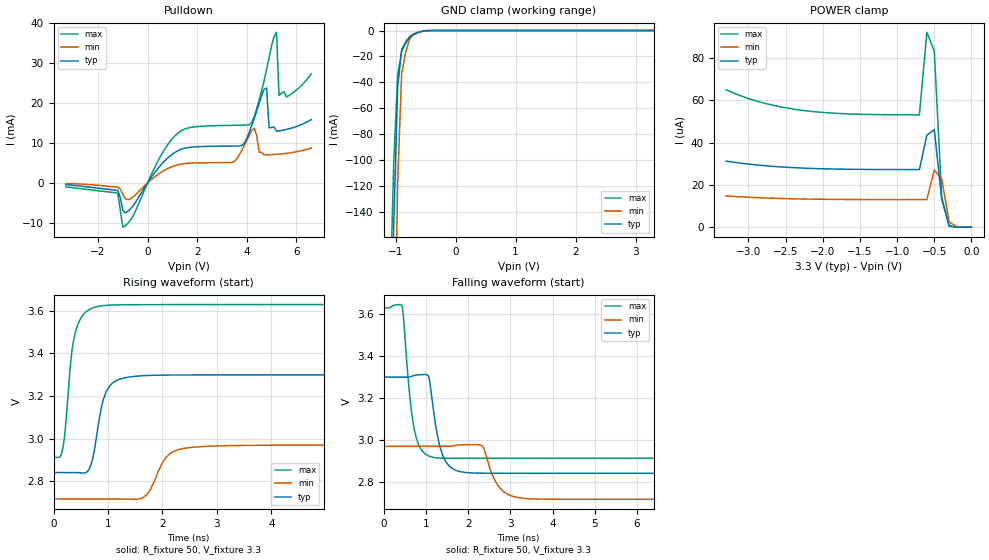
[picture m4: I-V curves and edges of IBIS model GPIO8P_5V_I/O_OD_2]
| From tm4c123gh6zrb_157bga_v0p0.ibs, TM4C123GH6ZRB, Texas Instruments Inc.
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|   Model Cell GPIO8P_5V_I/O_OD_2
[Model]   GPIO8P_5V_I/O_OD_2
Model_type   I/O_open_drain
Polarity   Inverting
Enable   Active-Low
Vinl =  0.8
Vinh =  2
Cref =  15.0000pF
Rref =  100.0000M
Vref =  0V
Vmeas =  1.65
C_comp   4.711578p   4.034737p   5.423069p
[Model Spec]
Vinl   0.8   0.8   0.8
Vinh   2   2   2
[Temperature Range]   25   125   -40
[Voltage Range]   3.3   2.97   3.63
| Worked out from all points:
|   slope of the pulldown table from 0 to 0.495 V, typ, clamps not added: 118 ohm
|   GND clamp passes 1 mA (typ) near -0.59 V on its own axis
|   rising waveform, R_fixture 50, V_fixture 3.3: 20-80 % time 209ps typ, 304ps min, 170ps max; typ from 2.84 V to 3.3 V
|   falling waveform, R_fixture 50, V_fixture 3.3: 20-80 % time 252ps typ, 337ps min, 213ps max; typ from 3.3 V to 2.84 V
| Nom Voltages:
|   VDDC=1.2, VDD=3.3, GND=0
| Min Voltages:
|   VDDC=1.08, VDD=2.97, GND=0
| Max Voltages:
|   VDDC=1.32, VDD=3.63, GND=0
[POWER_clamp]
|   voltage   I(typ)   I(min)   I(max)
-3.3V     31.22uA    14.76uA    64.95uA
-3.1V     30.25uA    14.33uA    62.09uA
-2.8V     29.13uA    13.84uA    58.77uA
-2.3V     27.98uA    13.34uA    55.36uA
-1.7V     27.4uA     13.1uA     53.62uA
-700mV    27.24uA    13.03uA    53.12uA
-600mV    43.52uA    13.03uA    92.14uA
-500mV    46.16uA    27.05uA    83.3uA
-400mV    13.21uA    22.74uA    13.98uA
-300mV    630.7nA    2.501uA    480.9nA
-200mV    23.21nA    190.8nA    10.65nA
0V        660.4pA    10.19nA    564.9pA
[Pulldown]
|   voltage   I(typ)   I(min)   I(max)
-3.3V     -450.7uA   -192.2uA   -1.006mA
-1.2V     -1.893mA   -1.109mA   -2.697mA
-1V       -6.866mA   -2.892mA   -11.1mA
1.2V      7.958mA    4.478mA    12.33mA
3.5V      9.211mA    5.381mA    14.4mA
4.2V      14.36mA    13.04mA    15.06mA
4.5V      19.92mA    7.668mA    20.83mA
4.8V      23.73mA    7.004mA    28.42mA
4.9V      13.75mA    7.03mA     31.35mA
5.2V      12.91mA    7.14mA     37.68mA
5.3V      13mA       7.19mA     21.9mA
6.6V      15.82mA    8.714mA    27.27mA
[GND_clamp]
|   voltage   I(typ)   I(min)   I(max)
-3.3V     -16.3A     -15.26A    -17.13A
-1.1V     -340.4mA   -570.5mA   -222.8mA
-1.033V   -152.7mA   -296.8mA   -103.3mA
-966.7mV  -44.18mA   -117.7mA   -34.4mA
-900mV    -14.77mA   -33.12mA   -16.14mA
-833.3mV  -8.752mA   -16.68mA   -9.833mA
-766.7mV  -4.716mA   -6.551mA   -5.563mA
-700mV    -2.657mA   -2.741mA   -3.333mA
-566.7mV  -672.8uA   -727.2uA   -724.4uA
-433.3mV  -51.87uA   -90.8uA    -37.79uA
3.3V      660.4pA    5.308uA    422.7pA
[Ramp]
| variable   typ   min   max
dV/dt_f 0.28269897/0.25386606n 0.15654957/0.33829046n 0.43992818/0.21519855n
dV/dt_r 0.38699946/0.53401128n 0.23880101/0.85366195n 0.55927105/0.38819382n
R_load = 50
[Rising Waveform]
R_fixture = 50
V_fixture = 3.3
V_fixture_min = 2.97
V_fixture_max = 3.63
|   time   V(typ)   V(min)   V(max)
0s        2.841V     2.717V     2.912V
178.1ps   2.841V     2.717V     2.965V
341.5ps   2.841V     2.717V     3.419V
428.4ps   2.841V     2.717V     3.523V
687.2ps   2.877V     2.717V     3.61V
833.7ps   3.083V     2.717V     3.622V
1.166ns   3.274V     2.717V     3.628V
2.143ns   3.299V     2.931V     3.63V
2.818ns   3.299V     2.964V     3.63V
20.12ns   3.3V       2.97V      3.63V
[Falling Waveform]
R_fixture = 50
V_fixture = 3.3
V_fixture_min = 2.97
V_fixture_max = 3.63
|   time   V(typ)   V(min)   V(max)
0s        3.3V       2.97V      3.63V
436.2ps   3.3V       2.97V      3.639V
720.2ps   3.308V     2.97V      3.054V
1.059ns   3.305V     2.97V      2.925V
1.179ns   3.141V     2.97V      2.917V
1.464ns   2.899V     2.97V      2.913V
2.039ns   2.843V     2.978V     2.913V
2.834ns   2.842V     2.755V     2.913V
3.318ns   2.841V     2.722V     2.913V
20.12ns   2.841V     2.717V     2.913V
